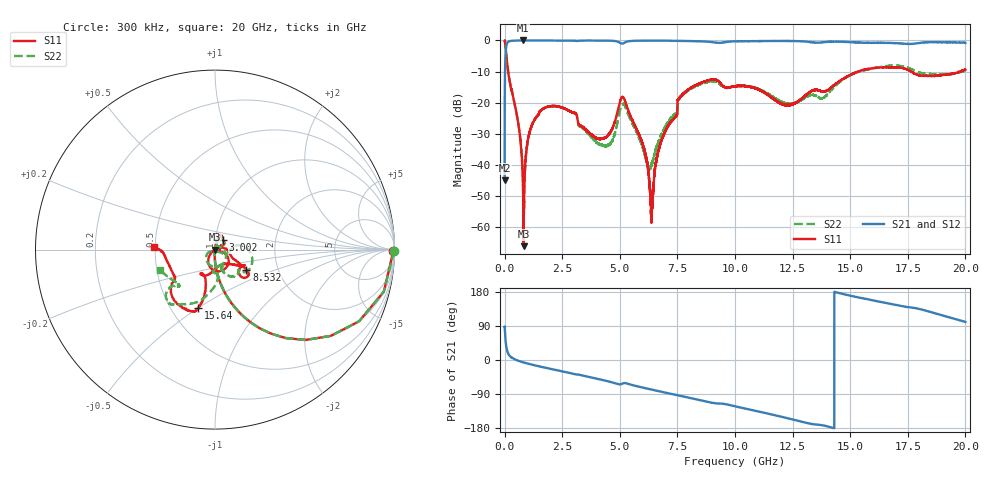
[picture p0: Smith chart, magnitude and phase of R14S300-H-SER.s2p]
!{R14S300}
!Johanson Technology Inc.
!www.johansontechnology.com
!Test Board Conditions:
!Substrate Type  RO4350B
!Substrate Thickness  20 mil
!Substrate Dk  3.66
!TL Type: GCPW
!TL Trace Width  36 mil
!TL Gap  12 mil
!Electrode orientation  Horizontal
!DUT TOPOLOGY	SERIES
!Mounting Pad LxW  26x36 mil
! Created Wed Nov 25 17:33:21 2020
! 2 Port Network Data from SP1.SP block
! freq  magS11  angS11  magS21  angS21  magS12  angS12  magS22  angS22
# khz S ma R 50
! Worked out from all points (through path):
!   20001 points, 300 kHz to 20 GHz, reference 50 ohm
!   highest |S21| = 0.00 dB at 779.3 MHz (marker M1); lowest = -45.0 dB at 300 kHz (marker M2)
!   group delay of S21, straight-line fit = 36 ps
!   lowest |S11| = -66.2 dB at 828.3 MHz (marker M3), VSWR 1.00, Z = 50 + j0.0168 ohm
!   |S11| at or under -10 dB: 154.3 MHz to 15.34 GHz (15.19 GHz wide, 196 % of centre); 17.64 GHz to 19.77 GHz (2.133 GHz wide, 11.4 % of centre); 19.77035 GHz to 19.77619 GHz (5.843 MHz wide, 0.0295 % of centre)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
!   |S22| runs from -58.3 to 0.0 dB; largest |S21 - S12| = 0.02
!   S11 on the Smith chart (normalised r, x): 300 kHz: open; 3.002 GHz: 1.09, +0.11; 8.532 GHz: 1.38, -0.32; 15.64 GHz: 0.68, -0.50; 20 GHz: 0.49, +0.02
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300  0.9933 -0.5  0.005616 88.4  0.005651 89.3  0.998 -0.5
128300  0.3763 -68.8  0.9251 21.1  0.9253 21.0  0.3776 -68.8
610300  0.0419 -92.4  0.999 -2.3  0.9978 -2.3  0.04225 -91.2
779300  0.007864 -99.3  0.9999 -5.6  0.999 -5.7  0.008344 -88.9
828300  0.0004888 159.8  0.9989 -6.5  0.9993 -6.5  0.001394 -22.9
1084300  0.03334 80.3  0.9983 -10.7  0.9977 -10.7  0.03291 76.3
1533300  0.07288 75.4  0.9958 -17.3  0.9962 -17.2  0.07269 69.7
3002300  0.06832 48.9  0.9927 -36.7  0.9918 -36.7  0.06816 50.9
3334300  0.04185 36.8  0.9947 -40.2  0.9953 -40.3  0.04034 51.9
4490300  0.03021 -18.9  0.9925 -56.2  0.9922 -56.2  0.02086 68.3
5158300  0.1208 -85.7  0.9005 -61.2  0.9003 -61.2  0.09526 -93.1
6029300  0.01937 -144.5  0.9915 -73.2  0.9915 -73.2  0.01691 -151.4
6375300  0.001638 117.7  0.9926 -78.1  0.9922 -78.0  0.009736 -70.4
6667300  0.01643 30.7  0.9931 -82.0  0.9927 -82.0  0.02336 -33.3
7600300  0.121 -26.7  0.9829 -94.2  0.9834 -94.2  0.1183 11.2
8532300  0.2076 -32.4  0.9664 -106.7  0.9656 -106.7  0.1996 -6.1
1.00003e7  0.1832 -28.6  0.9669 -122.1  0.9671 -122.1  0.1829 -43.9
1.22573e7  0.09116 -67.2  0.9801 -153.3  0.9825 -153.2  0.09651 -68.2
1.33343e7  0.154 -110.2  0.9361 -168.9  0.9375 -168.9  0.1324 -86.4
1.56403e7  0.3395 -105.8  0.9148 161.7  0.9244 161.8  0.3348 -115.7
1.66673e7  0.3672 -115.9  0.9146 149.1  0.9052 148.8  0.3909 -128.4
2e7  0.341 177.5  0.9163 100.5  0.917 100.7  0.3278 -160.2
